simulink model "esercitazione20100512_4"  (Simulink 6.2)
settings: Solver=FixedStepDiscrete  StartTime=0.0  StopTime=10  RelTol=1e-3
libraries: cstblocks x3

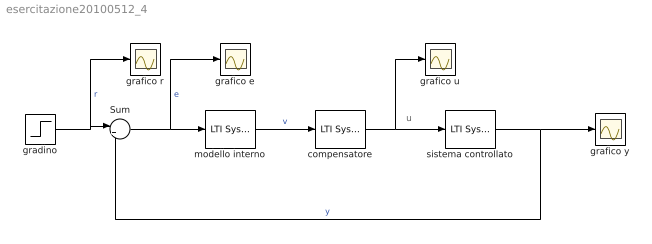
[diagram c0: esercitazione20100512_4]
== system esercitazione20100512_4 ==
  note: u
  Sum : Sum  Inputs=|+-
  compensatore : cstblocks/LTI System  sys=C  IC=0
  gradino : Step  Time=0  SampleTime=1
  grafico e : Scope
  grafico r : Scope
  grafico u : Scope
  grafico y : Scope
  modello interno : cstblocks/LTI System  sys=M  IC=0
  sistema controllato : cstblocks/LTI System  sys=P  IC=0
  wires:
  modello interno/1 -> compensatore/1  "v"
  compensatore/1 -> grafico u/1, sistema controllato/1
  Sum/1 -> grafico e/1, modello interno/1  "e"
  gradino/1 -> Sum/1, grafico r/1  "r"
  sistema controllato/1 -> grafico y/1, Sum/2  "y"
